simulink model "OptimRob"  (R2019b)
settings: Solver=VariableStepAuto  StartTime=0.0  StopTime=10.0  RelTol=1e-5
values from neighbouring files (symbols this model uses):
  Ki = 6.0    (= 6)    [EjemploOptimizRobusta.m]
  Kp = 6.9    [EjemploOptimizRobusta.m]
undefined symbols (not defined in the file or in its folder): d, tau
libraries: simulink x1

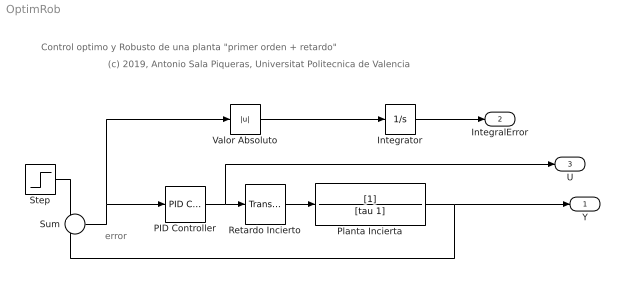
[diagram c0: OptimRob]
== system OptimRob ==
  note: (c) 2019, Antonio Sala Piqueras, Universitat Politecnica de Valencia
  note: Control optimo y Robusto de una planta "primer orden + retardo"
  note: error
  Integrator : Integrator
  PID Controller : simulink/Continuous/PID Controller  Controller=PID  Form=Parallel  TimeDomain=Continuous-time  SampleTime=-1  IntegratorMethod=Forward Euler  FilterMethod=Forward Euler  ControllerParametersSource=internal  P=Kp  I=Ki  D=0  UseFilter=on  N=100  TunerSelectOption=Transfer Function Based (PID Tuner App)  InitialConditionSource=internal  InitialConditionForIntegrator=0  InitialConditionForFilter=0  DifferentiatorICPrevScaledInput=0  ExternalReset=none  TrackingMode=off  Kt=1  LimitOutput=off  UpperSaturationLimit=inf  LowerSaturationLimit=-inf  LinearizeAsGain=on  AntiWindupMode=none  Kb=1  POutMin=[]  POutMax=[]  IOutMin=[]  IOutMax=[]  DOutMin=[]  DOutMax=[]  NOutMin=[]  NOutMax=[]  SumOutMin=[]  SumOutMax=[]  SaturationOutMin=[]  SaturationOutMax=[]  PParamMin=[]  PParamMax=[]  IParamMin=[]  IParamMax=[]  DParamMin=[]  DParamMax=[]  NParamMin=[]  NParamMax=[]  KbParamMin=[]  KbParamMax=[]  KtParamMin=[]  KtParamMax=[]  KbOutMin=[]  KbOutMax=[]  KtOutMin=[]  KtOutMax=[]  IntegratorOutMin=[]  IntegratorOutMax=[]  FilterOutMin=[]  FilterOutMax=[]  SumI1OutMin=[]  SumI1OutMax=[]  SumI2OutMin=[]  SumI2OutMax=[]  SumI3OutMin=[]  SumI3OutMax=[]  SumI4OutMin=[]  SumI4OutMax=[]  SumDOutMin=[]  SumDOutMax=[]  DifferentiatorOutMin=[]  DifferentiatorOutMax=[]  FilterDiffOutCoefMin=[]  FilterDiffOutCoefMax=[]  ReciprocalOutMin=[]  ReciprocalOutMax=[]  SumDenOutMin=[]  SumDenOutMax=[]  SumNumOutMin=[]  SumNumOutMax=[]  DivideOutMin=[]  DivideOutMax=[]  IntegratorContinuousStateAttributes=''  IntegratorStateMustResolveToSignalObject=off  IntegratorRTWStateStorageClass=Auto  FilterContinuousStateAttributes=''  FilterStateMustResolveToSignalObject=off  FilterRTWStateStorageClass=Auto  ParallelPVariant=InternalParameters  IdealPVariant=Disabled  IVariant=InternalParameters  DVariant=InternalParameters  IntegratorVariant=Continuous  SatVariant=Disabled  AWVariant=Passthrough  PCopyVariant=Disabled  TRVariant=Disabled  FdbkBlocksVariant=Forward  IdealPFdbkVariant=Disabled  SatFdbkVariant=Disabled  DerivativeFilterVariant=ContFilter  NVariant=InternalParameters  NCopyVariant=Disabled  FilterICVariant=InternalICsFilter  IntegratorICVariant=InternalICs  ExternalResetVariant=Disabled  TRSumVariant=Passthrough  SumFdbkVariant=Disabled  SumVariant=Sum_PID
  Planta Incierta : TransferFcn  Denominator=[tau 1]
  Retardo Incierto : TransportDelay  DelayTime=d
  Step : Step  Time=0  SampleTime=0
  Sum : Sum  Inputs=+-
  Valor Absoluto : Abs
  Y : Outport
  IntegralError : Outport  Port=2
  U : Outport  Port=3
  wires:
  Step/1 -> Sum/1
  Planta Incierta/1 -> Y/1, Sum/2
  Sum/1 -> Valor Absoluto/1, PID Controller/1
  Valor Absoluto/1 -> Integrator/1
  Integrator/1 -> IntegralError/1
  PID Controller/1 -> U/1, Retardo Incierto/1
  Retardo Incierto/1 -> Planta Incierta/1
